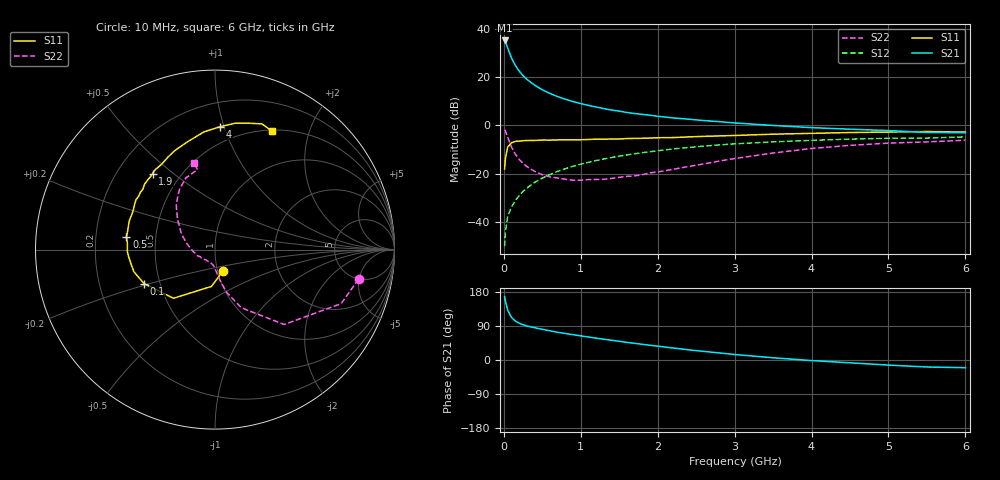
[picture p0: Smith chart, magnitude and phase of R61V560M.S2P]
! SIEMENS Small Signal Semiconductors
! BFR193
! Si NPN RF Bipolar Junction Transistor in SOT23
! VCE = 1.5 V  IC = 60 mA
! Common Emitter S-Parameters:  May  1996
# GHz  S  MA  R  50
!  f  S11  S21  S12  S22
! GHz  MAG  ANG  MAG  ANG  MAG  ANG  MAG  ANG
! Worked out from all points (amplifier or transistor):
!   36 points, 10 MHz to 6 GHz, reference 50 ohm
!   highest |S21| = 35.1 dB at 10 MHz (marker M1)
!   |S21| within 3 dB of that: start of sweep to 48.97 MHz
!   unconditionally stable (mu >= 1): 240.6 MHz to 2.279 GHz
!   at 250 MHz: K = 1.01, MAG = 23.5 dB, |S12| = -27.3 dB
!   at 1.4 GHz: K = 1.04, MAG = 8.6 dB, |S12| = -13.3 dB
!   at 6 GHz: K = 0.99, MSG = 0.9 dB, |S12| = -4.7 dB
!   S11 on the Smith chart (normalised r, x): 10 MHz: 1.06, -0.25; 100 MHz: 0.41, -0.19; 500 MHz: 0.34, +0.06; 1.9 GHz: 0.35, +0.42; 4 GHz: 0.38, +0.97; 6 GHz: 0.52, +1.47
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0.01  0.1261 -68.9  56.91 167.5  0.0032 76.5  0.817 -11.6
0.02  0.2061 -95.5  53.73 155.8  0.0062 76.4  0.7646 -23.2
0.05  0.3567 -130.5  39.88 131.5  0.0132 67.6  0.5679 -47.3
0.1  0.4381 -154.3  24.64 112.2  0.0207 68.8  0.3559 -65.6
0.15  0.4687 -164.8  17.26 102.6  0.0281 70.8  0.253 -74.1
0.2  0.475 -170.7  13.25 97.0  0.0356 72.6  0.1982 -78.4
0.25  0.4827 -175.3  10.68 92.9  0.0432 73.8  0.163 -81.8
0.3  0.4886 -178.7  8.951 89.9  0.0509 74.4  0.1411 -84.1
0.4  0.4892 175.9  6.786 85.2  0.0663 74.4  0.1125 -88.8
0.5  0.4988 171.7  5.454 80.9  0.0817 74.1  0.0956 -93.0
0.6  0.4974 167.9  4.567 77.0  0.0968 73.1  0.0867 -97.1
0.7  0.501 163.8  3.937 73.1  0.1123 72.2  0.0817 -101.6
0.9  0.503 157.4  3.109 66.9  0.1431 69.4  0.0736 -112.0
1.1  0.5118 151.6  2.592 60.6  0.173 66.7  0.0761 -121.4
1.4  0.5245 142.2  2.079 52.1  0.2172 61.9  0.0804 -136.4
1.9  0.5484 129.4  1.622 38.9  0.2865 53.7  0.1047 -161.7
2.2  0.5609 121.9  1.429 31.7  0.3258 48.6  0.1238 -175.7
3.5  0.659 95.3  0.998 5.9  0.4572 26.8  0.2695 140.9
4  0.6853 87.6  0.9 -1.5  0.4914 19.6  0.3334 130.5
4.5  0.7133 80.9  0.835 -7.4  0.521 12.6  0.3871 121.0
5.5  0.7478 69.5  0.715 -18.4  0.5483 -0.9  0.4566 102.3
6  0.7318 64.2  0.706 -20.3  0.5794 -4.9  0.4938 103.6
